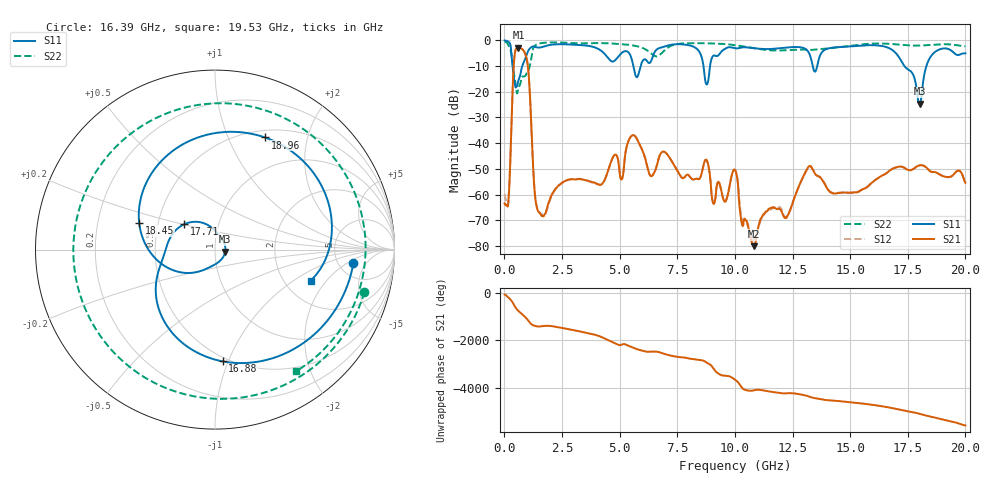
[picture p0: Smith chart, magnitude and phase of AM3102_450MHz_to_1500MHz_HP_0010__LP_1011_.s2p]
!Agilent Technologies,E8364B,MY43040894,A.07.50.67
!Agilent E8364B: A.07.50.67
!Date: Thursday, January 11, 2018 05:28:27
!Correction: S11(Full 2 Port(1,2))
!S21(Full 2 Port(1,2))
!S12(Full 2 Port(1,2))
!S22(Full 2 Port(1,2))
!S2P File: Measurements: S11, S21, S12, S22:
# Hz S  dB  R 50
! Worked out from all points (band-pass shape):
!   1601 points, 10 MHz to 20 GHz, reference 50 ohm
!   highest |S21| = -2.87 dB at 609.7 MHz (marker M1); lowest = -80.1 dB at 10.82 GHz (marker M2)
!   |S21| within 3 dB of the highest: 442.9 MHz to 926.4 MHz (483.5 MHz wide, 70.6 % of centre)
!   lowest |S11| = -24.7 dB at 18.01 GHz (marker M3), VSWR 1.12, Z = 56 - j1.31 ohm
!   |S11| at or under -10 dB: 356.7 MHz to 776.1 MHz (419.4 MHz wide, 74 % of centre); 5.594 GHz to 5.91 GHz (315.9 MHz wide, 5.49 % of centre); 17.35 GHz to 18.31 GHz (954.6 MHz wide, 5.35 % of centre)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
!   |S22| runs from -20.7 to -0.5 dB; largest |S21 - S12| = 0.0017
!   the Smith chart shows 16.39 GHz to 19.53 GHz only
!   S11 on the Smith chart (normalised r, x): 16.39 GHz: 6.93, -2.54; 16.88 GHz: 0.47, -0.95; 17.71 GHz: 0.68, +0.20; 18.45 GHz: 0.39, +0.14; 18.96 GHz: 0.58, +1.37; 19.53 GHz: 2.76, -1.40
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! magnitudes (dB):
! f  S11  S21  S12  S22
! 10 MHz  -0.1  -63.5  -59.8  -0.5
! 172.4 MHz  -0.6  -63.1  -62.6  -1.9
! 422.3 MHz  -15.2  -7.8  -7.8  -13.4
! 609.7 MHz  -15.6  -2.9  -2.9  -18.6
! 997 MHz  -4.8  -8.6  -8.6  -12.5
! 1.497 GHz  -2.8  -67.0  -66.6  -1.3
! 3.346 GHz  -1.9  -54.1  -54.0  -1.2
! 6.682 GHz  -3.2  -46.4  -46.3  -6.1
! 8.781 GHz  -17.2  -46.7  -46.7  -1.2
! 9.08 GHz  -5.9  -63.6  -63.5  -1.2
! 10.01 GHz  -3.1  -50.5  -50.4  -1.9
! 10.82 GHz  -3.1  -80.1  -77.8  -3.0
! 13.34 GHz  -8.6  -49.6  -49.6  -3.7
! 16.39 GHz  -2.2  -52.6  -52.7  -1.3
! 16.68 GHz  -3.0  -51.0  -50.9  -1.4
! 16.88 GHz  -4.1  -49.8  -49.8  -1.5
! 17.71 GHz  -13.0  -50.2  -50.3  -2.0
! 18.01 GHz  -24.7  -48.6  -48.6  -2.0
! 18.45 GHz  -7.0  -50.8  -50.8  -1.8
! 18.96 GHz  -3.3  -52.6  -52.5  -1.5
! 19.53 GHz  -5.0  -51.8  -51.8  -1.8
! 20 GHz  -5.1  -55.4  -55.7  -2.3
